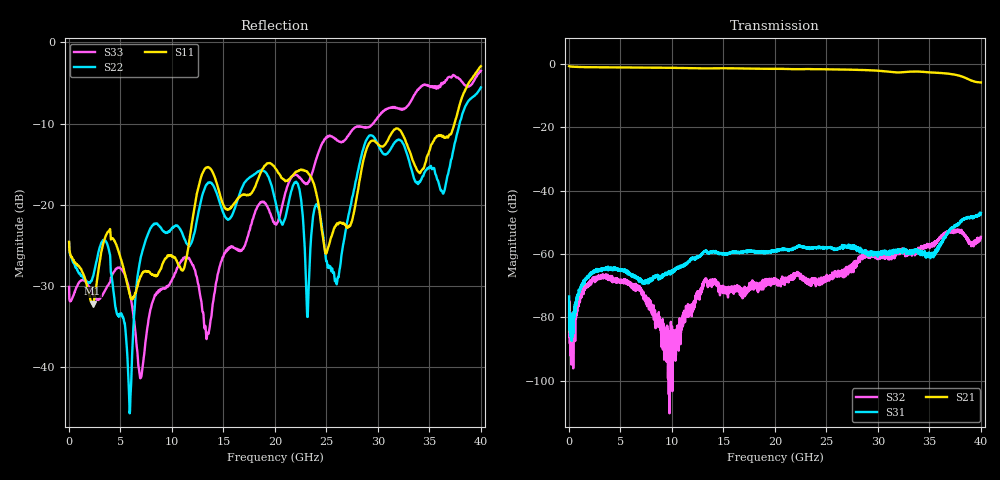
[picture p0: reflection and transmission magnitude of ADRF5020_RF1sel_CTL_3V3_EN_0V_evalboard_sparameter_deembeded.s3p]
! Device:  ADRF5020
! Description: SOI MMIC SPDT Non-Reflective Switch
! Frequency:  0.1 -  30 GHz
! Ports:
! 	RFC	= Port 1
!	RF1	= Port 2
!	RF2	= Port 3
! Vdd:  +3.3 Volt
! Vss:  -2.5 Volt
! Control:  0/+3.3 Volt
! State:  RF1 Selected (Vctl= 3.3 V, Ven= 0 V)
! Data:	Data was collected using a calibrated network analyzer with AFR software.
!	Fixtures were calculated using AFR and fixturing was applied to collect
!	this Deembedded  S Parameter data of ADRF5020.
! Note:	Analog Devices supplies this data as a sample of measured data at the package pin
!	for this product.  Your particular data for this product may vary.
!	Data was taken at 25 degrees C.
!	Analog Devices reserves the right to change this data at anytime.
# Hz S  dB  R 50
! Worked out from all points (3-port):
!   4000 points, 10 MHz to 40 GHz, reference 50 ohm
!   strongest paths, dB at 10 MHz, 10.01 GHz, 20.01 GHz, 30.01 GHz, 40 GHz:
!     S21: -0.7, -1.2, -1.5, -2.1, -5.8
!     S31: -73.4, -65.6, -59.1, -59.8, -47.0
!     S32: -79.5, -88.2, -68.4, -60.7, -54.6
!   lowest |S11| = -32.2 dB at 2.29 GHz (marker M1), VSWR 1.05, Z = 51.6 - j1.96 ohm
!   |S11| at or under -10 dB: start of sweep to 37.42 GHz
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1e7  -24.55 -5.4  -0.71 -0.5  -77.01 129.6
     -0.71 -0.5  -24.63 -4.6  -76.73 113.8
     -73.38 29.0  -79.49 -39.4  -30.09 146.6
2.29e9  -32.16 -50.3  -1.03 -27.6  -65.67 58.9
        -1.04 -27.5  -28.92 -51.6  -68.19 40.6
        -65.73 60.8  -67.92 44.0  -30.92 169.7
5.91e9  -31.06 -57.7  -1.12 -70.1  -66.42 41.6
        -1.12 -70.0  -45.51 -86.9  -70.06 -8.6
        -66.45 40.5  -68.91 -5.7  -30.83 -113.8
6.96e9  -28.78 -94.3  -1.15 -82.5  -68.28 52.3
        -1.15 -82.4  -26.49 -158.8  -70.67 -27.9
        -67.78 54.0  -71.31 -26.8  -41.23 -141.1
9.31e9  -26.63 -112.1  -1.20 -110.4  -66.47 92.8
        -1.21 -110.2  -23.35 -99.2  -95.53 -76.7
        -66.66 92.6  -88.27 -3.1  -30.25 -141.8
2.001e10  -15.44 -151.3  -1.54 121.8  -59.04 77.3
          -1.55 122.1  -19.30 -131.6  -68.72 -70.2
          -59.05 77.8  -68.37 -72.5  -22.33 -42.8
2.599e10  -22.36 -111.9  -1.74 45.9  -58.58 49.3
          -1.75 46.3  -29.76 -176.4  -66.16 170.9
          -58.43 50.1  -65.94 169.4  -12.00 -62.5
2.926e10  -12.23 -108.9  -1.98 3.6  -60.02 26.2
          -1.99 4.0  -11.44 -85.8  -60.00 132.9
          -59.73 27.9  -60.50 132.8  -10.31 -86.0
3.492e10  -13.64 -124.8  -2.64 -78.1  -60.37 30.6
          -2.64 -77.6  -15.44 -154.1  -57.37 15.8
          -60.52 28.6  -57.00 17.6  -5.36 -110.8
4e10  -2.92 -128.6  -5.83 -158.9  -47.26 24.2
      -5.84 -158.3  -5.53 -56.4  -54.93 -121.4
      -46.98 24.6  -54.57 -119.0  -3.50 -137.6
